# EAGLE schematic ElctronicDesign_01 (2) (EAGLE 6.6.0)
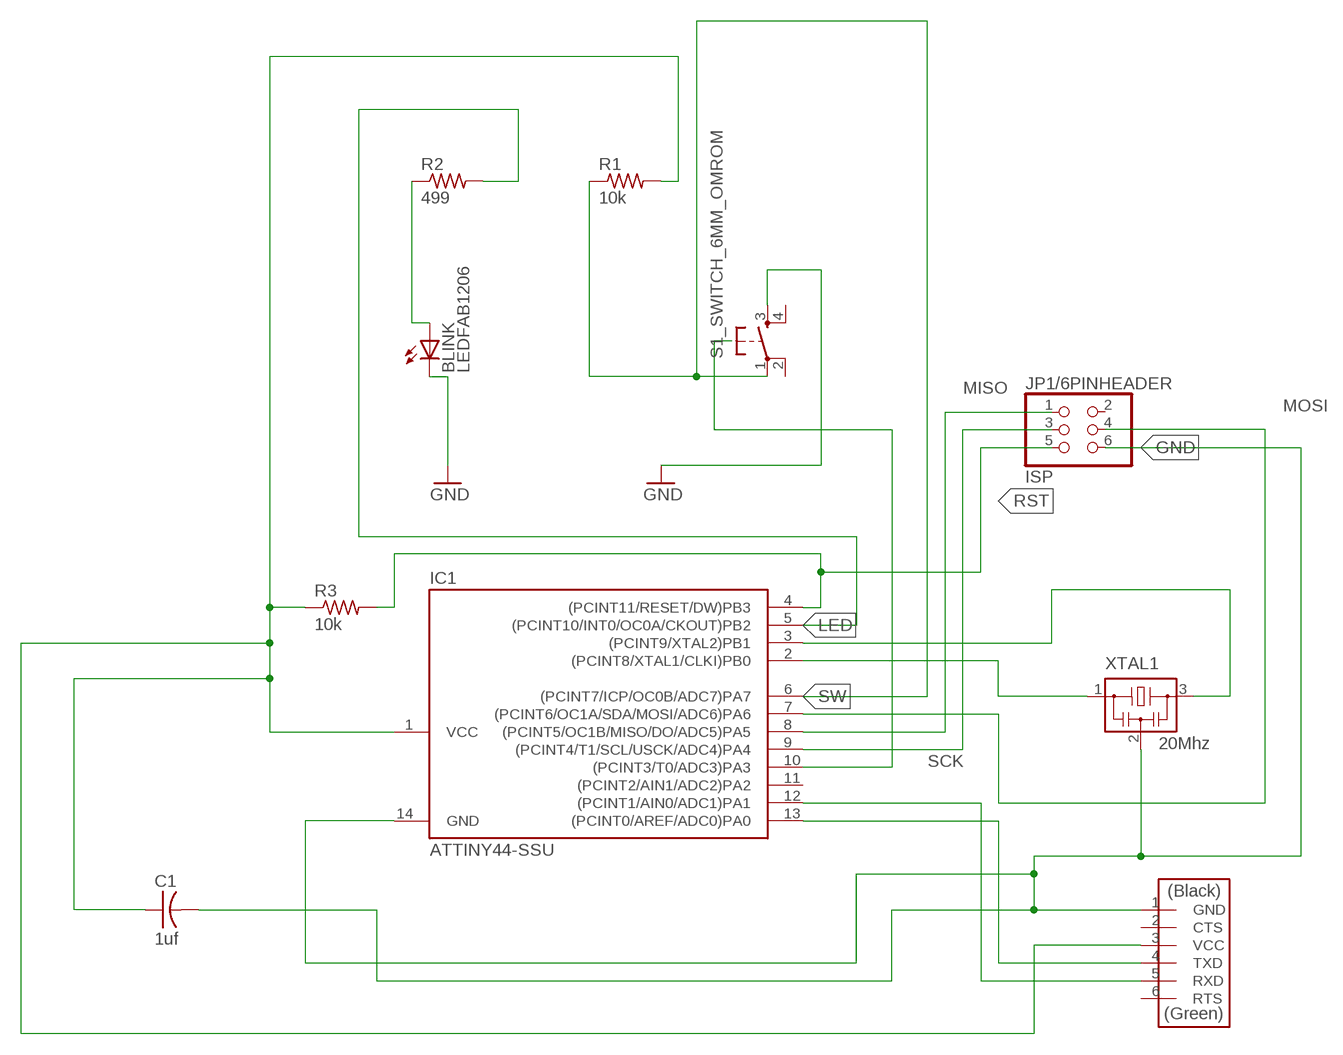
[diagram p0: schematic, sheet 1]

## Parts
BLINK  LEDFAB1206  [LED1206FAB]
C1  1uf  CAP-US1206FAB  [C1206FAB]
IC1  ATTINY44-SSU  [SOIC14]
J2_FTDI_HEADER  FTDI-SMD-HEADER  [1X06SMD]
JP1/6PINHEADER  ISP  PINHD-2X3-SMD  [2X03SMD]
R1  10k  RES-US1206FAB  [R1206FAB]
R2  499  RES-US1206FAB  [R1206FAB]
R3  10k  RES-US1206FAB  [R1206FAB]
S1_SWITCH_6MM_OMROM  6MM_SWITCH6MM_SWITCH  [6MM_SWITCH]
XTAL1  20Mhz  RESONATOR  [EFOBM]

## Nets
GND: BLINK.2(C) C1.2 IC1.14(GND) J2_FTDI_HEADER.1(GND) JP1/6PINHEADER.6 S1_SWITCH_6MM_OMROM.3(S) XTAL1.2
JUNTION: R1.1 S1_SWITCH_6MM_OMROM.1(P)
LED: IC1.5((PCINT10/INT0/OC0A/CKOUT)PB2) R2.2
MISO: IC1.8((PCINT5/OC1B/MISO/DO/ADC5)PA5) JP1/6PINHEADER.1
MOSI: IC1.7((PCINT6/OC1A/SDA/MOSI/ADC6)PA6) JP1/6PINHEADER.4
N$1: BLINK.1(A) R2.1
N$2: IC1.3((PCINT9/XTAL2)PB1) XTAL1.3
N$4: IC1.2((PCINT8/XTAL1/CLKI)PB0) XTAL1.1
N$5: IC1.10((PCINT3/T0/ADC3)PA3)
N$6: IC1.12((PCINT1/AIN0/ADC1)PA1) J2_FTDI_HEADER.5(RXD)
N$7: IC1.13((PCINT0/AREF/ADC0)PA0) J2_FTDI_HEADER.4(TXD)
N$8: C1.1 IC1.1(VCC) J2_FTDI_HEADER.3(VCC) R1.2 R3.1
RST: IC1.4((PCINT11/RESET/DW)PB3) JP1/6PINHEADER.5 R3.2
SCK: IC1.9((PCINT4/T1/SCL/USCK/ADC4)PA4) JP1/6PINHEADER.3
SW: IC1.6((PCINT7/ICP/OC0B/ADC7)PA7)
Unconnected: IC1.11((PCINT2/AIN1/ADC2)PA2) J2_FTDI_HEADER.2(CTS) J2_FTDI_HEADER.6(RTS) JP1/6PINHEADER.2 S1_SWITCH_6MM_OMROM.2(P1) S1_SWITCH_6MM_OMROM.4(S1)

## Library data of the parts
BLINK = fab:LED: LED
C1 = fab:CAP-US
IC1 = fab:ATTINY44
J2_FTDI_HEADER = fab:FTDI-SMD-HEADER
JP1/6PINHEADER = fab:PINHD-2X3-SMD: PIN HEADER
R1-R3 = fab:RES-US: Resistor (US Symbol)
S1_SWITCH_6MM_OMROM = fab:6MM_SWITCH: OMRON SWITCH
XTAL1 = fab:RESONATOR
